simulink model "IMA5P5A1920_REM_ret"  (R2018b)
settings: Solver=VariableStepAuto  StartTime=0  StopTime=10.0  RelTol=1e-3
InitFcn:
  | %% Matlab program: InitIMA5A1920P5.m
  | %Matlab init file for REM IMA5A1920P5
  | clc; clear
  | 
  | %%Batterie
  | BAT.U = 9 ;%tension de la pile en V
  | 
  | 
  | %%Regulateur 5V
  | 
  | RED.UBAT = 5/9; % regulateur de tension 5V
  | 
  | 
  | %%Cellule photovoltaïque
  | 
  | PV.I0 = 1; %courant de saturation, fluctue avec l'irradiance sur la cellule
  | PV.VT = 8.2; %tension en court circuit
  | PV.k = 1.3806e-23; %constante de Boltzmann en J.K-1
  | PV.q = 1.6022e-19; %charge d'un electrion en C
  | PV.TC = 18;
  | PV.T = PV.TC + 273.15; %température en Kelvin
  | %%MPPT
  | 
  | 
  | 
  | %%Moteur courant continu
  |     % --- MCC Parameters ---
  |         % --- Description ---
  | 
  |     MCC.U = 1.5;							% Nominal voltage of the armature winding (V)
  |     MCC.I = 0.190;							% Nominal Current of the armature winding (A)
  |     MCC.N = 8200;								% Nominal speed (rpm)
  |     MCC.W = MCC.N*pi/30;					% Nominal speed (rad/s)
  |     MCC.P = MCC.U*MCC.I;    % Nominal electrical power of the armature winding (W)
  |     MCC.P_util = 0.4;                          % Nominal useful power (W)
  |     MCC.tho = 0.003;
  |     MCC.Kphi = 0.0018;
  |     MCC.R=1;
  |     MCC.L=0.184;
  | 
  | %%Véhicule
  | 
  | VEH.R = 0.0145;%rayon de la roue en m
  | 
  | VEH.M = 0.467; %masse du mobile en kg
  | 
  | VEH.MPLUS = 0; %masse en charge sur le véhicule en kg
  | 
  | VEH.MTOT = VEH.M + VEH.MPLUS; %masse totale du véhicule
  | 
  | VEH.J = 0.05; %inertie du véhicule à définir
  | 
  | VEH.f = 0.05; %frottements
  | 
  | 	    % --- Electromechanical conversion ---
  | 
  |       % Torque Coefficient via the excitation Flux
  |     MCC.K  = MCC.W /MCC.U;
  |     MCC.tho = 0.0014;
  | 
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libraries: simulink x2

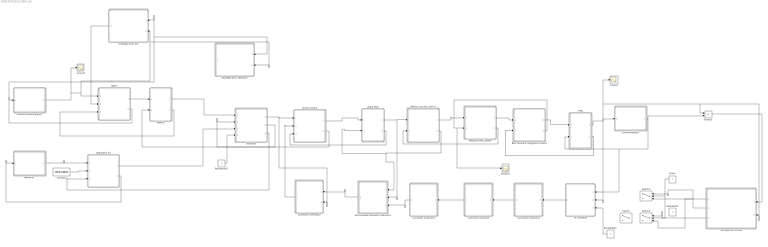
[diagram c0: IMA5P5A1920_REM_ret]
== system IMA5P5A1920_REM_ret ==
  Accumulation element inversion1 : Subsystem  AncestorBlock=simulink/SMC/Asservissement Correcteur IP
  Batterie7 : Subsystem  AncestorBlock=simulink/REM/SE
  Bloc fusionné (vispignon+roues) : Subsystem  AncestorBlock=simulink/REM/EC Elec  mask(Hacheur){}
  Cellule photovoltaïque7 : Subsystem  AncestorBlock=simulink/REM/SE
  "Choix " : Constant  Commented=on
  Constant : Constant  Value=RED.UBAT
  Converter inversion : Subsystem  AncestorBlock=simulink/SMC/Inversion EC avec mesure
  Converter inversion1 : Subsystem  AncestorBlock=simulink/SMC/Inversion EC avec mesure
  Converter inversion2 : Subsystem  AncestorBlock=simulink/SMC/Inversion EC avec mesure
  Converter inversion3 : Subsystem  AncestorBlock=simulink/SMC/Inversion EC avec mesure
  Driver moteur : Subsystem  AncestorBlock=simulink/REM/EC Elec  mask(Hacheur){}
  Environnement : Subsystem  AncestorBlock=simulink/REM/SE
  Induit MCC : Subsystem  AncestorBlock=simulink/REM/EA  mask(CM){}
  MPPT : Subsystem  AncestorBlock=simulink/REM/EC Elec  mask(Hacheur){}
  MPPT2 : Subsystem  AncestorBlock=simulink/REM/EA  mask(CM){}
  Moteur courant continu : Subsystem  AncestorBlock=simulink/REM/EC EM
  PFD : Subsystem  AncestorBlock=simulink/REM/EA  mask(CM){}
  PI controller : Subsystem  AncestorBlock=simulink/SMC/Asservissement Correcteur IP
  Product : Product
  Reduction MCC/arbre : Subsystem  AncestorBlock=simulink/REM/EC Elec  mask(Hacheur){}
  Rentabilité : Constant  Commented=on
  Rentabilité1 : Constant
  Rentabilité2 : Constant
  Selecteur : Subsystem  mask(CM){}
  Strategie de vitesse : Subsystem  Commented=on  AncestorBlock=simulink/SMC/Inversion EC avec mesure
  Strategie pour kr2 : Subsystem  Commented=on  AncestorBlock=simulink/SMC/Inversion EC avec mesure
  Strategie pour selecteur : Subsystem  Commented=on  AncestorBlock=simulink/SMC/Inversion EC avec mesure
  Switch : Switch  Criteria=u2 ~= 0
  Switch1 : Switch  Commented=on  Threshold=2
  Switch2 : Switch  Commented=on  Criteria=u2 ~= 0
  courant : Scope
  regulateur 5V : Subsystem  AncestorBlock=simulink/REM/EC Elec  mask(Hacheur){}
  vitesse : Scope
  vitesse1 : Scope
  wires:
  Selecteur/1(Usel) -> Driver moteur/1(Usel), Converter inversion3/2(u_sel)
  Induit MCC/2(Iind) -> Driver moteur/3(Iind)
  Driver moteur/1(Udriver) -> Induit MCC/1(Udriver)
  Induit MCC/1(I_ind) -> Accumulation element inversion1/2(I_ind), Moteur courant continu/1(I_ind)
  Driver moteur/2(Idriver) -> Selecteur/2(Idriver)
  Moteur courant continu/2(UMCC) -> Induit MCC/2(UMCC), Accumulation element inversion1/1(UMCC)
  Reduction MCC/arbre/2(OmegaMCC) -> Moteur courant continu/2(OmegaMCC)
  Moteur courant continu/1(TMCC) -> Reduction MCC/arbre/1(TMCC)
  MPPT/2(Uint) -> Strategie pour kr2/1(Upv), Strategie pour selecteur/1(Upv), Cellule photovoltaïque7/1(Uint)
  MPPT/1(Imppt) -> MPPT2/1(Imppt)
  MPPT2/2(U_mppt) -> MPPT/3(Umppt)
  MPPT2/1(Umppt) -> Selecteur/1(Umppt)
  Constant/1 -> regulateur 5V/2(mreg)
  Batterie7/1(Ubat) -> regulateur 5V/1(Ubat)
  regulateur 5V/2(Ibat) -> Batterie7/1(Ibat)
  regulateur 5V/1(U5v) -> Selecteur/3(Ubatt)
  Selecteur/2(Isel1) -> MPPT2/2(Isel1)
  Selecteur/3(Isel2) -> regulateur 5V/3(Isel2)
  Reduction MCC/arbre/1(Tred) -> Bloc fusionné (vispignon+roues)/1(Tred)
  Bloc fusionné (vispignon+roues)/1(Tred2) -> PFD/1(Tred2)
  PFD/1(v_vehicule) -> Environnement/1(V_vehicule), PI controller/2(V_vehicule), Strategie de vitesse/2(v_vehicule), Product/1, vitesse/1
  Environnement/1(F_res) -> PI controller/1(F_res), PFD/2(Fres), Product/2
  PFD/2(vvehicule) -> Bloc fusionné (vispignon+roues)/2(v_vehicule)
  PI controller/1(Tred2_ref) -> Converter inversion1/1(Tred_2_ref)
  Strategie pour kr2/1(mh) -> MPPT/2(mh)
  Converter inversion3/1(reg_uP) -> Driver moteur/2(reg_uP)
  Accumulation element inversion1/1(u_driver_ref) -> Converter inversion3/1(u_driver_ref)
  Converter inversion2/1(I_ind_ref) -> Accumulation element inversion1/3(I_ind_ref)
  Converter inversion/1(T_MCC_ref) -> Converter inversion2/1(T_MCC_ref)
  Converter inversion1/1(Tred_ref) -> Converter inversion/1(T_red_ref)
  Product/1 -> Strategie de vitesse/1(P_trac)
  Strategie de vitesse/3(v_rapidité) -> Switch1/1
  "Choix "/1 -> Switch2/2, Switch1/2
  Strategie de vitesse/1(v_vehicule_rampe) -> Switch1/3, Switch2/1
  Strategie de vitesse/2(v_vehicule_rendement) -> Switch2/3
  Rentabilité1/1 -> PI controller/3(V_vehicule_ref)
  Cellule photovoltaïque7/1(Ipv) -> courant/1, Strategie pour selecteur/2(Ipv), Strategie pour kr2/2(Ipv), MPPT/1(Ipv)
  Rentabilité2/1 -> Selecteur/4(selecteur)
  Bloc fusionné (vispignon+roues)/2(Omega_arbre) -> vitesse1/1, Reduction MCC/arbre/2(Omega)

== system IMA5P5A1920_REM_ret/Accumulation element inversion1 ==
  UMCC : Inport
  I_ind : Inport  Port=2
  I_ind_ref : Inport  Port=3
  PI Controller : Subsystem
  the sign depends of the relationships of the model1 : Sum
  u_driver_ref : Outport  InitialOutput=0
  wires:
  PI Controller/1(I_ref) -> the sign depends of the relationships of the model1/2
  the sign depends of the relationships of the model1/1 -> u_driver_ref/1
  UMCC/1 -> the sign depends of the relationships of the model1/1
  I_ind/1 -> PI Controller/1(I_ind_ref)
  I_ind_ref/1 -> PI Controller/2(I_ind)

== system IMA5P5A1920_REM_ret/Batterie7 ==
  Ibat : Inport
  Constant : Constant  Value=9
  Scope : Scope
  Ubat : Outport  InitialOutput=0
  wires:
  Constant/1 -> Ubat/1
  Ibat/1 -> Scope/1

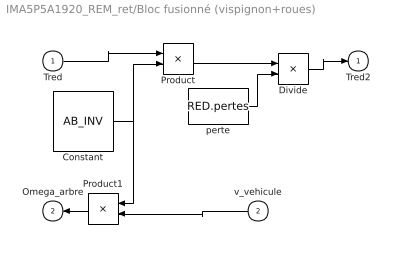
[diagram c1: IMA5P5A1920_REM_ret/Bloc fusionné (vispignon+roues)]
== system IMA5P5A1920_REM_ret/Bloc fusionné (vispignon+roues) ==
  Tred : Inport
  v_vehicule : Inport  Port=2
  Constant : Constant  Value=AB_INV
  Divide : Product  Inputs=*/
  Product : Product
  Product1 : Product
  perte : Constant  Value=RED.pertes
  Tred2 : Outport  InitialOutput=0
  Omega_arbre : Outport  Port=2  InitialOutput=0
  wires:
  Tred/1 -> Product/1
  Product/1 -> Divide/1
  Product1/1 -> Omega_arbre/1
  v_vehicule/1 -> Product1/2
  Constant/1 -> Product1/1, Product/2
  perte/1 -> Divide/2
  Divide/1 -> Tred2/1

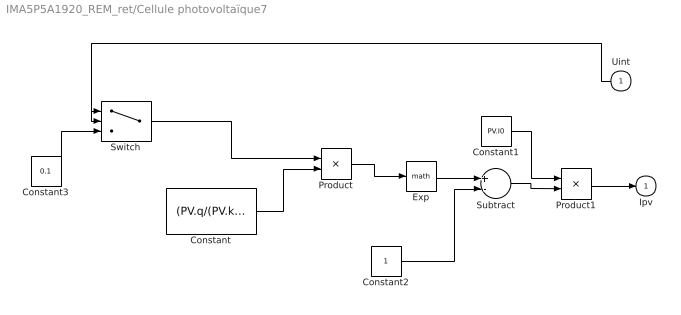
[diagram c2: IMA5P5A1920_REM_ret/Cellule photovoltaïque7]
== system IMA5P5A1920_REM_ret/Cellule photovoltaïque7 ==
  Uint : Inport
  Constant : Constant  Value=(PV.q/(PV.k*PV.T))
  Constant1 : Constant  Value=PV.I0
  Constant2 : Constant
  Constant3 : Constant  Value=0.1
  Exp : Math
  Product : Product
  Product1 : Product
  Subtract : Sum  Inputs=+-
  Switch : Switch  Criteria=u2 > Threshold
  Ipv : Outport  InitialOutput=0
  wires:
  Product1/1 -> Ipv/1
  Uint/1 -> Switch/2, Switch/1
  Constant/1 -> Product/2
  Product/1 -> Exp/1
  Exp/1 -> Subtract/1
  Constant2/1 -> Subtract/2
  Subtract/1 -> Product1/2
  Constant1/1 -> Product1/1
  Constant3/1 -> Switch/3
  Switch/1 -> Product/1

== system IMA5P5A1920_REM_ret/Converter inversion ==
  T_red_ref : Inport
  Constant : Constant  Value=RED.VP
  Divide : Product  Inputs=*/
  T_MCC_ref : Outport  InitialOutput=0
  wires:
  Divide/1 -> T_MCC_ref/1
  Constant/1 -> Divide/2
  T_red_ref/1 -> Divide/1

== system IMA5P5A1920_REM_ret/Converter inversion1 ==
  Tred_2_ref : Inport
  Constant : Constant  Value=AB_INV
  Divide : Product  Inputs=*/
  Product : Product
  perte : Constant  Value=RED.pertes
  Tred_ref : Outport  InitialOutput=0
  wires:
  Constant/1 -> Divide/2
  Tred_2_ref/1 -> Product/1
  perte/1 -> Product/2
  Product/1 -> Divide/1
  Divide/1 -> Tred_ref/1

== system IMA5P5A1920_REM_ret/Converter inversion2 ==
  T_MCC_ref : Inport
  Constant : Constant  Value=MCC.K
  Divide : Product  Inputs=*/
  I_ind_ref : Outport  InitialOutput=0
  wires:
  T_MCC_ref/1 -> Divide/1
  Constant/1 -> Divide/2
  Divide/1 -> I_ind_ref/1

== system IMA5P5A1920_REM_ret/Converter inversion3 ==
  u_driver_ref : Inport
  u_sel : Inport  Port=2
  Divide : Product  Inputs=*/
  reg_uP : Outport  InitialOutput=0
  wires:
  u_driver_ref/1 -> Divide/1
  u_sel/1 -> Divide/2
  Divide/1 -> reg_uP/1

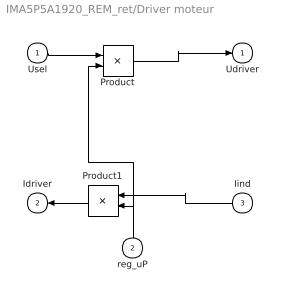
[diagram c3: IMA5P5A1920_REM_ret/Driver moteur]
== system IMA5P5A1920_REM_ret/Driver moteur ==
  Usel : Inport
  reg_uP : Inport  Port=2
  Iind : Inport  Port=3
  Product : Product
  Product1 : Product
  Udriver : Outport  InitialOutput=0
  Idriver : Outport  Port=2  InitialOutput=0
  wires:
  reg_uP/1 -> Product1/2, Product/2
  Usel/1 -> Product/1
  Product/1 -> Udriver/1
  Iind/1 -> Product1/1
  Product1/1 -> Idriver/1

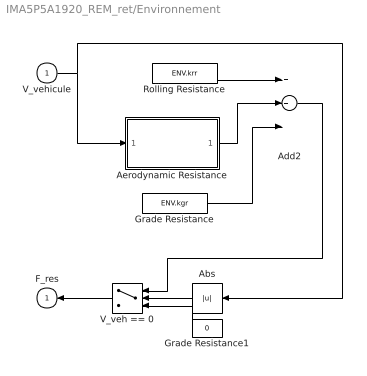
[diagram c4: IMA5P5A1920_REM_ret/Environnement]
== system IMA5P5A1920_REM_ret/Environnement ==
  V_vehicule : Inport
  Abs : Abs
  Add2 : Sum  Inputs=3
  Aerodynamic Resistance : Subsystem
  Grade Resistance : Constant  Value=ENV.kgr
  Grade Resistance1 : Constant  Value=0
  Rolling Resistance : Constant  Value=ENV.krr
  V_veh == 0 : Switch  Threshold=0.1
  F_res : Outport  InitialOutput=0
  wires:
  Grade Resistance1/1 -> V_veh == 0/3
  Abs/1 -> V_veh == 0/2
  Rolling Resistance/1 -> Add2/1
  Aerodynamic Resistance/1(F_ar) -> Add2/2
  V_veh == 0/1 -> F_res/1
  Grade Resistance/1 -> Add2/3
  Add2/1 -> V_veh == 0/1
  V_vehicule/1 -> Aerodynamic Resistance/1(V_veh), Abs/1

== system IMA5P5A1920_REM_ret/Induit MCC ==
  Udriver : Inport
  UMCC : Inport  Port=2
  Subtract : Sum  Inputs=+-
  Transfer Fcn : TransferFcn  Denominator=[MCC.L MCC.R]
  I_ind : Outport  InitialOutput=0
  Iind : Outport  Port=2  InitialOutput=0
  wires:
  Udriver/1 -> Subtract/1
  UMCC/1 -> Subtract/2
  Transfer Fcn/1 -> Iind/1, I_ind/1
  Subtract/1 -> Transfer Fcn/1

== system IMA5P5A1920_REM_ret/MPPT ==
  Ipv : Inport
  mh : Inport  Port=2
  Umppt : Inport  Port=3
  Product : Product
  Product1 : Product
  Imppt : Outport  InitialOutput=0
  Uint : Outport  Port=2  InitialOutput=0
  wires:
  mh/1 -> Product/2, Product1/2
  Ipv/1 -> Product/1
  Umppt/1 -> Product1/1
  Product1/1 -> Uint/1
  Product/1 -> Imppt/1

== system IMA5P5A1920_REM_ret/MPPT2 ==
  Imppt : Inport
  Isel1 : Inport  Port=2
  Subtract : Sum  Inputs=+-
  Transfer Fcn : TransferFcn  Denominator=[0.033 1]
  Umppt : Outport  InitialOutput=0
  U_mppt : Outport  Port=2  InitialOutput=0
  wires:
  Imppt/1 -> Subtract/1
  Isel1/1 -> Subtract/2
  Subtract/1 -> Transfer Fcn/1
  Transfer Fcn/1 -> U_mppt/1, Umppt/1

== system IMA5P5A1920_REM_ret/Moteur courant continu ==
  I_ind : Inport
  OmegaMCC : Inport  Port=2
  Constant : Constant  Value=MCC.Kphi
  Product : Product
  Product1 : Product
  TMCC : Outport  InitialOutput=0
  UMCC : Outport  Port=2  InitialOutput=0
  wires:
  I_ind/1 -> Product/1
  Constant/1 -> Product1/1, Product/2
  Product/1 -> TMCC/1
  OmegaMCC/1 -> Product1/2
  Product1/1 -> UMCC/1

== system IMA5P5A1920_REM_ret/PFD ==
  Tred2 : Inport
  Fres : Inport  Port=2
  Subtract : Sum  Inputs=+-
  Transfer Fcn : TransferFcn  Numerator=[AB2]  Denominator=[(VEH.J+VEH.MPLUS*AB2) VEH.f]
  v_vehicule : Outport  InitialOutput=0
  vvehicule : Outport  Port=2  InitialOutput=0
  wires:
  Fres/1 -> Subtract/2
  Tred2/1 -> Subtract/1
  Subtract/1 -> Transfer Fcn/1
  Transfer Fcn/1 -> vvehicule/1, v_vehicule/1

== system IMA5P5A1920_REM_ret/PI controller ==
  F_res : Inport
  V_vehicule : Inport  Port=2
  V_vehicule_ref : Inport  Port=3
  " " : Sum  Inputs=-+
  PI Controller : Subsystem
  Tred2_ref : Outport  InitialOutput=0
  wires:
  " "/1 -> Tred2_ref/1
  PI Controller/1(epsi) -> " "/2
  V_vehicule/1 -> PI Controller/1(V_chassis)
  V_vehicule_ref/1 -> PI Controller/2(V_chassis_ref)
  F_res/1 -> " "/1

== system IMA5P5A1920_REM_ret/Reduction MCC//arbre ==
  TMCC : Inport
  Omega : Inport  Port=2
  Constant : Constant  Value=RED.VP
  Product : Product
  Product1 : Product
  Tred : Outport  InitialOutput=0
  OmegaMCC : Outport  Port=2  InitialOutput=0
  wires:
  TMCC/1 -> Product/1
  Product/1 -> Tred/1
  Product1/1 -> OmegaMCC/1
  Omega/1 -> Product1/2
  Constant/1 -> Product/2, Product1/1

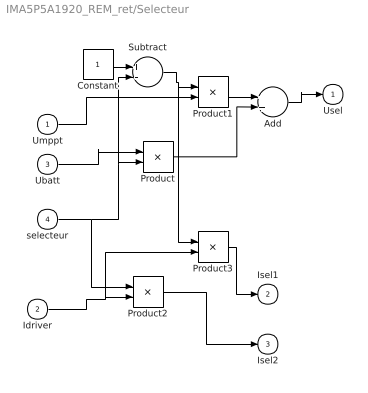
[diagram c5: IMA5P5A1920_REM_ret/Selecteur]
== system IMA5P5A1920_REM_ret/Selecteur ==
  Umppt : Inport
  Idriver : Inport  Port=2
  Ubatt : Inport  Port=3
  selecteur : Inport  Port=4
  Add : Sum
  Constant : Constant
  Product{,1..3} (4 alike) : Product
  Subtract : Sum  Inputs=+-
  Usel : Outport  InitialOutput=0
  Isel1 : Outport  Port=2  InitialOutput=0
  Isel2 : Outport  Port=3  InitialOutput=0
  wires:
  Ubatt/1 -> Product/1
  selecteur/1 -> Product2/1, Subtract/2, Product/2
  Constant/1 -> Subtract/1
  Umppt/1 -> Product1/2
  Subtract/1 -> Product3/1, Product1/1
  Product/1 -> Add/2
  Product1/1 -> Add/1
  Add/1 -> Usel/1
  Idriver/1 -> Product3/2, Product2/2
  Product2/1 -> Isel2/1
  Product3/1 -> Isel1/1

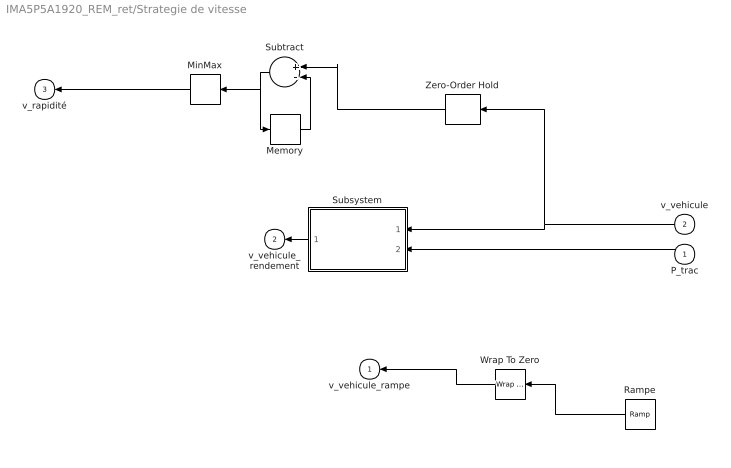
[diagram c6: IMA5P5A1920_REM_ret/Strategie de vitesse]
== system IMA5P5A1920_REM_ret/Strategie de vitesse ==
  P_trac : Inport
  v_vehicule : Inport  Port=2
  Memory : Memory
  MinMax : MinMax  Function=max
  Rampe : simulink/Sources/Ramp  slope=1  start=0  InitialOutput=0
  Subsystem : Subsystem
  Subtract : Sum  Inputs=+-
  Wrap To Zero : simulink/Discontinuities/Wrap To Zero  Threshold=10
  Zero-Order Hold : ZeroOrderHold  SampleTime=-1
  v_vehicule_rampe : Outport  InitialOutput=0
  v_vehicule_rendement : Outport  Port=2  InitialOutput=0
  v_rapidité : Outport  Port=3  InitialOutput=0
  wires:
  Wrap To Zero/1 -> v_vehicule_rampe/1
  Rampe/1 -> Wrap To Zero/1
  Subsystem/1(V_vehicule_ref2) -> v_vehicule_rendement/1
  P_trac/1 -> Subsystem/2(P_trac)
  v_vehicule/1 -> Zero-Order Hold/1, Subsystem/1(V_vehicule)
  Zero-Order Hold/1 -> Subtract/1
  Subtract/1 -> MinMax/1, Memory/1
  Memory/1 -> Subtract/2
  MinMax/1 -> v_rapidité/1

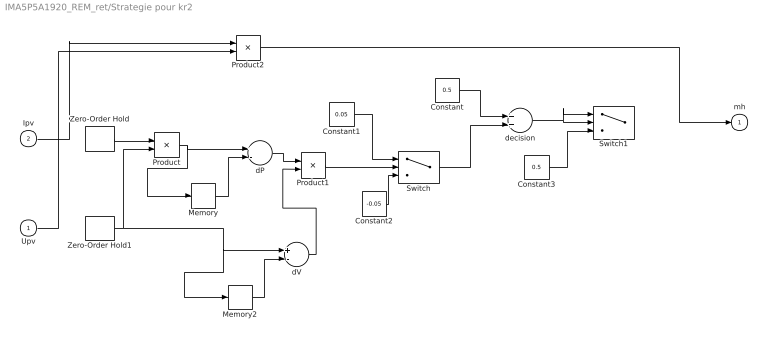
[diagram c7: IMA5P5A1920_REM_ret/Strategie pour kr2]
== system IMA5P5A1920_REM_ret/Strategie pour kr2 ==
  Upv : Inport
  Ipv : Inport  Port=2
  Constant : Constant  Commented=on  Value=0.5
  Constant1 : Constant  Commented=on  Value=0.05
  Constant2 : Constant  Commented=on  Value=-0.05
  Constant3 : Constant  Commented=on  Value=0.5
  Memory : Memory  Commented=on
  Memory2 : Memory  Commented=on
  Product : Product  Commented=on
  Product1 : Product  Commented=on
  Product2 : Product
  Switch : Switch  Commented=on
  Switch1 : Switch  Commented=on  Criteria=u2 > Threshold
  Zero-Order Hold : ZeroOrderHold  Commented=on  SampleTime=-1
  Zero-Order Hold1 : ZeroOrderHold  Commented=on  SampleTime=-1
  dP : Sum  Commented=on  Inputs=+-
  dV : Sum  Commented=on  Inputs=+-
  decision : Sum  Commented=on
  mh : Outport  InitialOutput=0
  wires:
  Zero-Order Hold/1 -> Product/1
  Memory/1 -> dP/2
  Ipv/1 -> Product2/1
  Upv/1 -> Product2/2
  Constant/1 -> decision/1
  Zero-Order Hold1/1 -> Memory2/1, dV/1, Product/2
  Memory2/1 -> dV/2
  dP/1 -> Product1/1
  dV/1 -> Product1/2
  Product1/1 -> Switch/2
  Constant1/1 -> Switch/1
  Constant2/1 -> Switch/3
  Switch/1 -> decision/2
  decision/1 -> Switch1/1, Switch1/2
  Constant3/1 -> Switch1/3
  Product/1 -> Memory/1, dP/1
  Product2/1 -> mh/1

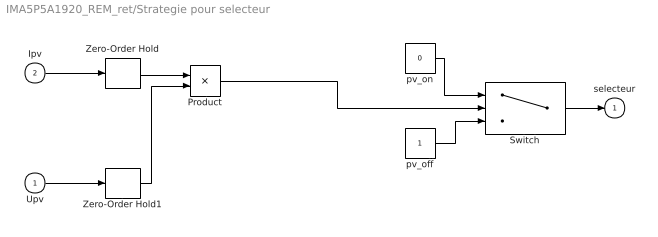
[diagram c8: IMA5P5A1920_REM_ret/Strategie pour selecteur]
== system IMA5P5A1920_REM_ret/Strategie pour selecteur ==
  Upv : Inport
  Ipv : Inport  Port=2
  Product : Product
  Switch : Switch  Threshold=0.4
  Zero-Order Hold : ZeroOrderHold  SampleTime=-1
  Zero-Order Hold1 : ZeroOrderHold  SampleTime=-1
  pv_off : Constant
  pv_on : Constant  Value=0
  selecteur : Outport  InitialOutput=0
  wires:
  Zero-Order Hold/1 -> Product/1
  Ipv/1 -> Zero-Order Hold/1
  Upv/1 -> Zero-Order Hold1/1
  Zero-Order Hold1/1 -> Product/2
  Product/1 -> Switch/2
  pv_on/1 -> Switch/1
  pv_off/1 -> Switch/3
  Switch/1 -> selecteur/1

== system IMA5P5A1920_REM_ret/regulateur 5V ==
  Ubat : Inport
  mreg : Inport  Port=2
  Isel2 : Inport  Port=3
  Product : Product
  Product1 : Product
  U5v : Outport  InitialOutput=0
  Ibat : Outport  Port=2  InitialOutput=0
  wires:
  mreg/1 -> Product1/2, Product/2
  Ubat/1 -> Product/1
  Product/1 -> U5v/1
  Isel2/1 -> Product1/1
  Product1/1 -> Ibat/1

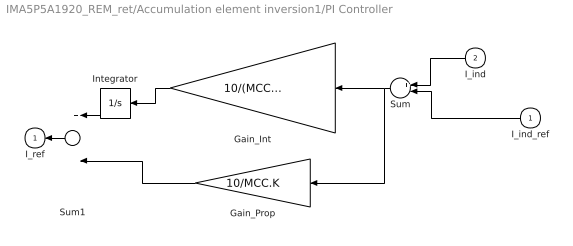
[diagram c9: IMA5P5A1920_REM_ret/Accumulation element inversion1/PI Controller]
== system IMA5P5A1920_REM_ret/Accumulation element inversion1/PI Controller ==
  I_ind_ref : Inport
  I_ind : Inport  Port=2
  Gain_Int : Gain  Gain=10/(MCC.K*MCC.tho)
  Gain_Prop : Gain  Gain=10/MCC.K
  Integrator : Integrator
  Sum : Sum  Inputs=+-
  Sum1 : Sum
  I_ref : Outport  InitialOutput=0
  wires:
  I_ind/1 -> Sum/1
  I_ind_ref/1 -> Sum/2
  Gain_Prop/1 -> Sum1/2
  Sum1/1 -> I_ref/1
  Integrator/1 -> Sum1/1
  Gain_Int/1 -> Integrator/1
  Sum/1 -> Gain_Prop/1, Gain_Int/1

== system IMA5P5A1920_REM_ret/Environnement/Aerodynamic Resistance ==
  V_veh : Inport
  Add1 : Sum
  Constant2 : Constant  Value=ENV.Vwind
  Gain3 : Gain  Gain=ENV.kaero
  Product : Product
  F_ar : Outport  InitialOutput=0
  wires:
  Gain3/1 -> F_ar/1
  Product/1 -> Gain3/1
  Add1/1 -> Product/1, Product/2
  Constant2/1 -> Add1/2
  V_veh/1 -> Add1/1

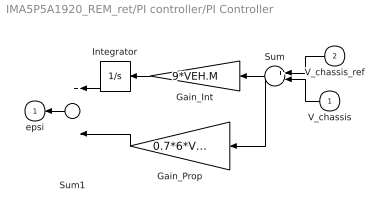
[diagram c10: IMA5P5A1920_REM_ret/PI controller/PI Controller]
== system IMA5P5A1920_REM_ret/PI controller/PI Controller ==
  V_chassis : Inport
  V_chassis_ref : Inport  Port=2
  Gain_Int : Gain  Gain=9*VEH.M
  Gain_Prop : Gain  Gain=0.7*6*VEH.M
  Integrator : Integrator
  Sum : Sum  Inputs=+-
  Sum1 : Sum
  epsi : Outport  InitialOutput=0
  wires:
  Sum/1 -> Gain_Prop/1, Gain_Int/1
  Gain_Int/1 -> Integrator/1
  Integrator/1 -> Sum1/1
  Sum1/1 -> epsi/1
  Gain_Prop/1 -> Sum1/2
  V_chassis/1 -> Sum/2
  V_chassis_ref/1 -> Sum/1

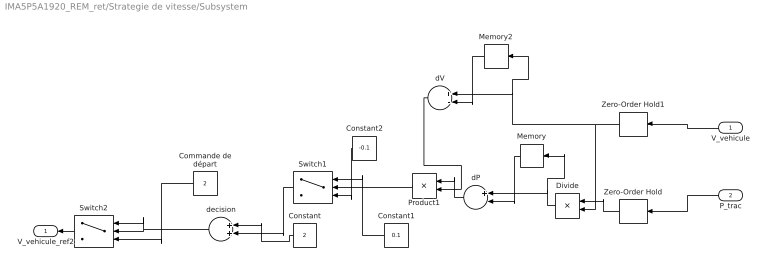
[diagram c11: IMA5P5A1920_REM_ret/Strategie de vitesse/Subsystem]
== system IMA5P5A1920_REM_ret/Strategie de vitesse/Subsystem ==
  V_vehicule : Inport
  P_trac : Inport  Port=2
  Commande de départ : Constant  Value=2
  Constant : Constant  Value=2
  Constant1 : Constant  Value=0.1
  Constant2 : Constant  Value=-0.1
  Divide : Product  Inputs=*/
  Memory : Memory
  Memory2 : Memory
  Product1 : Product
  Switch1 : Switch
  Switch2 : Switch  Criteria=u2 > Threshold
  Zero-Order Hold : ZeroOrderHold  SampleTime=-1
  Zero-Order Hold1 : ZeroOrderHold  SampleTime=-1
  dP : Sum  Inputs=+-
  dV : Sum  Inputs=+-
  decision : Sum
  V_vehicule_ref2 : Outport
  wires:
  Memory2/1 -> dV/2
  P_trac/1 -> Zero-Order Hold/1
  Constant2/1 -> Switch1/3
  Memory/1 -> dP/2
  Zero-Order Hold/1 -> Divide/1
  Zero-Order Hold1/1 -> Divide/2, Memory2/1, dV/1
  Divide/1 -> Memory/1, dP/1
  Commande de départ/1 -> Switch2/3
  decision/1 -> Switch2/1, Switch2/2
  Constant1/1 -> Switch1/1
  Constant/1 -> decision/1
  Switch1/1 -> decision/2
  dV/1 -> Product1/2
  Product1/1 -> Switch1/2
  dP/1 -> Product1/1
  Switch2/1 -> V_vehicule_ref2/1
  V_vehicule/1 -> Zero-Order Hold1/1
